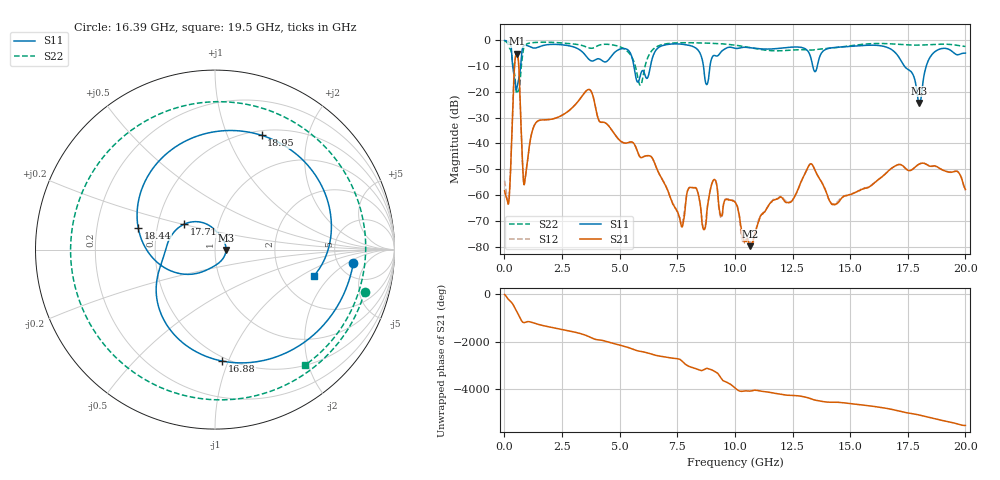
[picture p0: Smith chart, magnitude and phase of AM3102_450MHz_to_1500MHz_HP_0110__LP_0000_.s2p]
!Agilent Technologies,E8364B,MY43040894,A.07.50.67
!Agilent E8364B: A.07.50.67
!Date: Thursday, January 11, 2018 05:44:37
!Correction: S11(Full 2 Port(1,2))
!S21(Full 2 Port(1,2))
!S12(Full 2 Port(1,2))
!S22(Full 2 Port(1,2))
!S2P File: Measurements: S11, S21, S12, S22:
# Hz S  dB  R 50
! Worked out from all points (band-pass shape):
!   1601 points, 10 MHz to 20 GHz, reference 50 ohm
!   highest |S21| = -5.15 dB at 534.7 MHz (marker M1); lowest = -79.8 dB at 10.67 GHz (marker M2)
!   |S21| within 3 dB of the highest: 457.8 MHz to 610.8 MHz (153.1 MHz wide, 28.6 % of centre)
!   lowest |S11| = -24.3 dB at 18 GHz (marker M3), VSWR 1.13, Z = 56.5 - j0.164 ohm
!   |S11| at or under -10 dB: 361.3 MHz to 704.2 MHz (342.9 MHz wide, 64.4 % of centre); 5.618 GHz to 6.337 GHz (718.9 MHz wide, 12 % of centre); 17.35 GHz to 18.3 GHz (949.6 MHz wide, 5.33 % of centre)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
!   |S22| runs from -20.7 to -0.3 dB; largest |S21 - S12| = 0.0023
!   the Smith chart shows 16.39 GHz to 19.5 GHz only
!   S11 on the Smith chart (normalised r, x): 16.39 GHz: 6.93, -2.52; 16.88 GHz: 0.47, -0.95; 17.71 GHz: 0.68, +0.20; 18.44 GHz: 0.39, +0.12; 18.95 GHz: 0.55, +1.34; 19.5 GHz: 3.03, -1.31
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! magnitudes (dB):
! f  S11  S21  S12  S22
! 10 MHz  -0.1  -58.3  -54.4  -0.3
! 209.9 MHz  -0.8  -61.1  -59.6  -2.8
! 534.7 MHz  -18.7  -5.1  -5.1  -20.7
! 884.6 MHz  -1.9  -54.7  -54.7  -2.1
! 1.372 GHz  -2.9  -31.9  -31.9  -0.8
! 3.346 GHz  -4.2  -21.9  -21.9  -1.9
! 5.895 GHz  -13.7  -45.3  -45.3  -17.4
! 6.682 GHz  -2.8  -51.1  -51.2  -2.2
! 7.694 GHz  -1.5  -72.3  -70.7  -1.0
! 10.01 GHz  -3.1  -62.7  -62.6  -1.9
! 10.67 GHz  -2.9  -79.8  -78.7  -2.9
! 13.34 GHz  -8.4  -48.1  -48.0  -3.8
! 14.28 GHz  -2.8  -63.6  -63.6  -2.9
! 16.39 GHz  -2.2  -52.9  -52.8  -1.2
! 16.68 GHz  -3.0  -50.5  -50.5  -1.3
! 16.88 GHz  -4.1  -49.2  -49.1  -1.4
! 17.71 GHz  -13.1  -50.0  -50.0  -1.9
! 18 GHz  -24.3  -48.0  -48.0  -1.9
! 18.44 GHz  -7.0  -48.7  -48.8  -1.7
! 18.95 GHz  -3.2  -50.0  -50.0  -1.5
! 19.5 GHz  -4.9  -50.9  -50.9  -1.8
! 20 GHz  -5.0  -57.8  -58.3  -2.4
